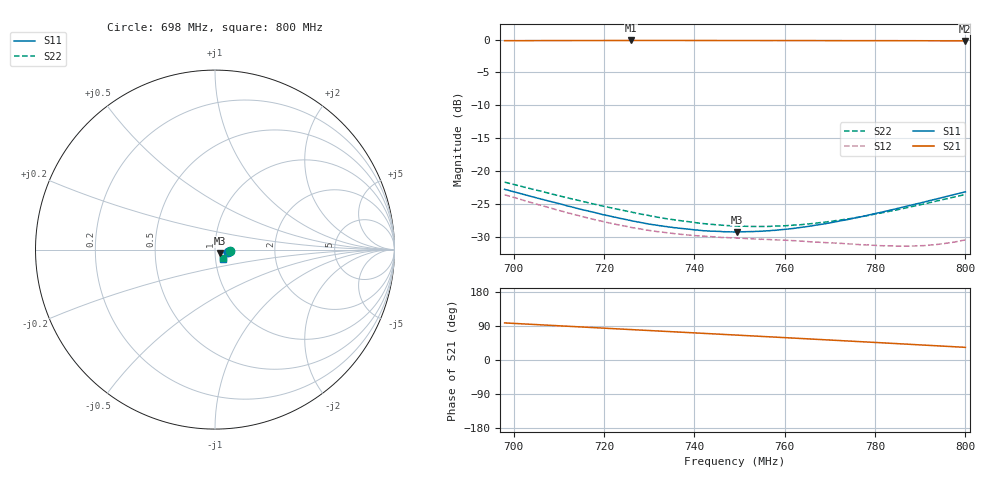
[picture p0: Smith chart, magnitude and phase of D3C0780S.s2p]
! 11/3/2020 1:38:03 PM
! C:\USERS\DITOM\DESKTOP\SINGLE JUNTION ISOLATOR DATA\0.698-800 MHZ (D3I0780S).S2P
! CHANNEL.1
! TR.MEASUREMENT
! CORRECTED.DATA
# GHZ S RI R 50.0
! FREQ.GHZ  S11RE  S11IM  S21RE  S21IM  S12RE  S12IM  S22RE  S22IM
!; PortSelection: Port_12
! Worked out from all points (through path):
!   601 points, 698 MHz to 800 MHz, reference 50 ohm
!   highest |S21| = -0.14 dB at 726 MHz (marker M1); lowest = -0.2 dB at 799.8 MHz (marker M2)
!   lowest |S11| = -29.3 dB at 749.5 MHz (marker M3), VSWR 1.07, Z = 52.7 - j2.25 ohm
!   |S11| at or under -10 dB: start of sweep to end of sweep
!   |S22| runs from -28.4 to -21.7 dB; largest |S21 - S12| = 1
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0.698  0.0717 -0.0122  -0.1348 0.9707  0.0631 -0.0191  0.0819 -0.00937
0.70667  0.0587 -0.0147  -0.0409 0.981  0.0458 -0.0287  0.0682 -0.0124
0.715  0.0483 -0.0164  0.0491 0.9817  0.0301 -0.0338  0.0572 -0.0147
0.72044  0.0428 -0.017  0.1073 0.9776  0.0205 -0.0352  0.0511 -0.0157
0.72605  0.0379 -0.0178  0.1669 0.9698  0.0116 -0.0354  0.0458 -0.0165
0.732  0.0338 -0.0186  0.229 0.9568  0.00318 -0.0344  0.041 -0.0174
0.73795  0.0307 -0.0195  0.2901 0.9397  -0.00409 -0.0325  0.0372 -0.0181
0.74203  0.0288 -0.0201  0.3313 0.9257  -0.00829 -0.0309  0.0352 -0.0187
0.749  0.027 -0.0214  0.4005 0.8974  -0.014 -0.0277  0.0326 -0.0197
0.74951  0.0269 -0.0213  0.4054 0.895  -0.0143 -0.0274  0.0326 -0.0199
0.75461  0.0264 -0.0227  0.4545 0.8707  -0.0173 -0.0248  0.0316 -0.0208
0.75818  0.0264 -0.0237  0.4883 0.8522  -0.019 -0.0232  0.0314 -0.0217
0.76192  0.0266 -0.0252  0.5227 0.831  -0.0201 -0.0217  0.0314 -0.0227
0.766  0.0274 -0.0268  0.5595 0.8062  -0.0209 -0.02  0.0318 -0.024
0.76957  0.0283 -0.0284  0.5908 0.7835  -0.0213 -0.019  0.0324 -0.0254
0.77433  0.0297 -0.0311  0.6311 0.7511  -0.0213 -0.018  0.0336 -0.0275
0.783  0.0336 -0.0371  0.7 0.686  -0.0204 -0.0176  0.0371 -0.0324
0.78759  0.036 -0.041  0.7339 0.6487  -0.0196 -0.0183  0.0394 -0.0357
0.7915  0.0384 -0.0447  0.7613 0.6153  -0.0189 -0.0195  0.0415 -0.0388
0.79626  0.0413 -0.0496  0.7927 0.5723  -0.0181 -0.0218  0.0445 -0.0433
0.79983  0.0435 -0.0538  0.8147 0.5388  -0.0178 -0.024  0.0467 -0.0469
0.8  0.0436 -0.0541  0.8158 0.5372  -0.0178 -0.0241  0.0468 -0.0469
